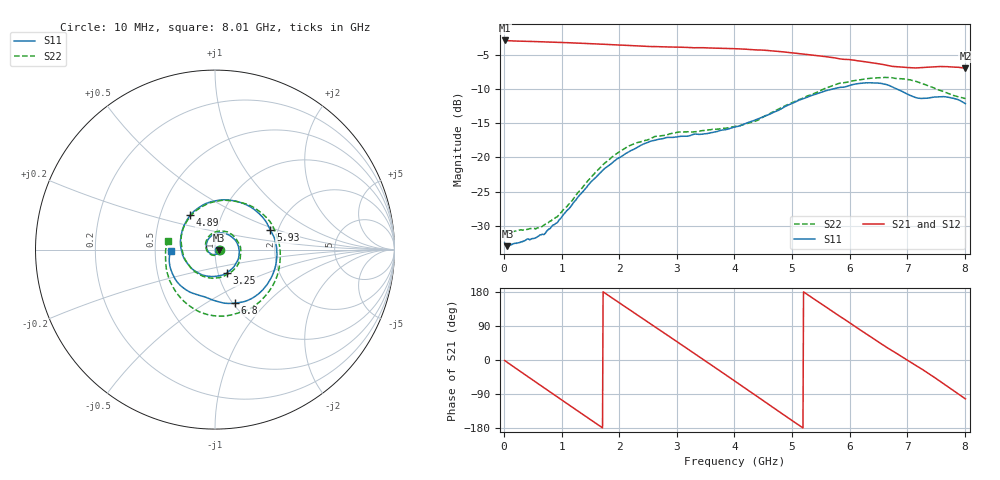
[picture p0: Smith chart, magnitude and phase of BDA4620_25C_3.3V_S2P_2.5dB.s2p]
!Agilent Technologies,E5071B,MY42404982,A.09.10
!Date: Wed May 06 08:56:29 2026
!Data & Calibration Information:
!Freq	S11:SOLT2(ON)	S21:SOLT2(ON)	S12:SOLT2(ON)	S22:SOLT2(ON)
# Hz S RI R 50
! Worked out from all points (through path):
!   801 points, 10 MHz to 8.01 GHz, reference 50 ohm
!   highest |S21| = -2.94 dB at 10 MHz (marker M1); lowest = -7.0 dB at 8.01 GHz (marker M2)
!   group delay of S21, straight-line fit = 285 ps
!   lowest |S11| = -32.9 dB at 60 MHz (marker M3), VSWR 1.05, Z = 52.3 - j0.322 ohm
!   |S11| at or under -10 dB: start of sweep to 5.718 GHz; 6.812 GHz to end of sweep
!   |S22| runs from -31.0 to -8.3 dB; largest |S21 - S12| = 0.003
!   S11 on the Smith chart (normalised r, x): 10 MHz: 1.05, -0.00; 3.25 GHz: 1.10, -0.29; 4.89 GHz: 0.71, +0.29; 5.93 GHz: 1.82, +0.45; 6.8 GHz: 1.02, -0.68; 8.01 GHz: 0.60, -0.01
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1e7  0.0237 -0.00168  0.7124 -0.0153  0.7132 -0.0155  0.0295 -0.00194
6e7  0.0223 -0.00308  0.7049 -0.0816  0.7065 -0.0829  0.0281 -0.00364
3.6e8  0.0179 -0.0171  0.5521 -0.4345  0.5526 -0.4357  0.0216 -0.0201
7.3e8  -0.00682 -0.0277  0.1556 -0.6774  0.1555 -0.6783  -0.00654 -0.0321
1.03e9  -0.0356 -0.0137  -0.2166 -0.6527  -0.2177 -0.6532  -0.0382 -0.0164
1.35e9  -0.0482 0.027  -0.5339 -0.4208  -0.5343 -0.4212  -0.0528 0.0277
1.64e9  -0.0274 0.0697  -0.6643 -0.0955  -0.6652 -0.0959  -0.0328 0.075
1.93e9  0.0219 0.0926  -0.615 0.2454  -0.6163 0.2463  0.0198 0.1028
2.32e9  0.0979 0.0669  -0.3053 0.5751  -0.3064 0.576  0.1032 0.0767
2.68e9  0.1353 -0.00926  0.0964 0.6342  0.0974 0.6351  0.143 0.00204
3.25e9  0.067 -0.1291  0.5823 0.2452  0.5836 0.2443  0.0845 -0.128
3.62e9  -0.0266 -0.1497  0.6052 -0.1655  0.6058 -0.1668  -0.0167 -0.1595
4.01e9  -0.1292 -0.105  0.3466 -0.5142  0.3467 -0.5152  -0.1294 -0.1077
4.44e9  -0.1916 0.0233  -0.115 -0.596  -0.1158 -0.5964  -0.1873 0.0313
4.89e9  -0.1389 0.1908  -0.4981 -0.3084  -0.4983 -0.3085  -0.1134 0.21
5.35e9  0.0603 0.2777  -0.5354 0.1501  -0.5359 0.1507  0.0999 0.2709
5.93e9  0.3086 0.1094  -0.1388 0.4995  -0.1385 0.5009  0.3432 0.0773
6.27e9  0.3377 -0.0901  0.1641 0.4707  0.1649 0.471  0.3532 -0.1206
6.68e9  0.1764 -0.2853  0.4036 0.2328  0.4053 0.2331  0.2057 -0.3229
6.8e9  0.1098 -0.2982  0.4346 0.149  0.4361 0.1485  0.1354 -0.3511
7.36e9  -0.1038 -0.2503  0.3741 -0.2581  0.3748 -0.2593  -0.1808 -0.2799
8.01e9  -0.2466 -0.00507  -0.097 -0.4367  -0.0977 -0.4381  -0.2645 0.0451
